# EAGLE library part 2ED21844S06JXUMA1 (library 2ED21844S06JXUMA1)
INFINEON - 2ED21844S06JXUMA1 - MOSFET DRIVER, -40 TO 125DEG C Source: Datasheet
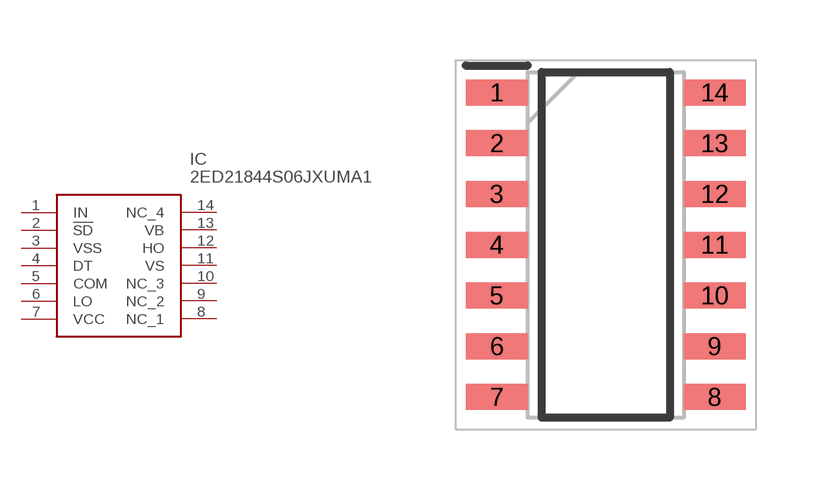
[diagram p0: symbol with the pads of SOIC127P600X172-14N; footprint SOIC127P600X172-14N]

Designator prefix IC

## 2ED21844S06JXUMA1 (Arrow_Part_Number: 2ED21844S06JXUMA1; Arrow_Price-Stock: https://www.arrow.com/en/products/2ed21844s06jxuma1/infineon-technologies-ag?region=nac; Description: INFINEON - 2ED21844S06JXUMA1 - MOSFET DRIVER, -40 TO 125DEG C; Height: 1.72mm; Manufacturer_Name: Infineon; Manufacturer_Part_Number: 2ED21844S06JXUMA1; Mouser_Part_Number: 726-2ED21844S06JXUMA; Mouser_Price-Stock: https://www.mouser.co.uk/ProductDetail/Infineon-Technologies/2ED21844S06JXUMA1?qs=BJlw7L4Cy7%252B8cvb7Sbexog%3D%3D)  [SOIC127P600X172-14N]
1  IN
2  !SD
3  VSS
4  DT
5  COM
6  LO
7  VCC
8  NC_1
9  NC_2
10  NC_3
11  VS
12  HO
13  VB
14  NC_4

## Footprint SOIC127P600X172-14N (pad centres in mm)
DSO - 14
smd 1.55 x 0.65: 1 -2.725,3.81; 2 -2.725,2.54; 3 -2.725,1.27; 4 -2.725,0; 5 -2.725,-1.27; 6 -2.725,-2.54; 7 -2.725,-3.81; 8 2.725,-3.81; 9 2.725,-2.54; 10 2.725,-1.27; 11 2.725,0; 12 2.725,1.27; 13 2.725,2.54; 14 2.725,3.81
